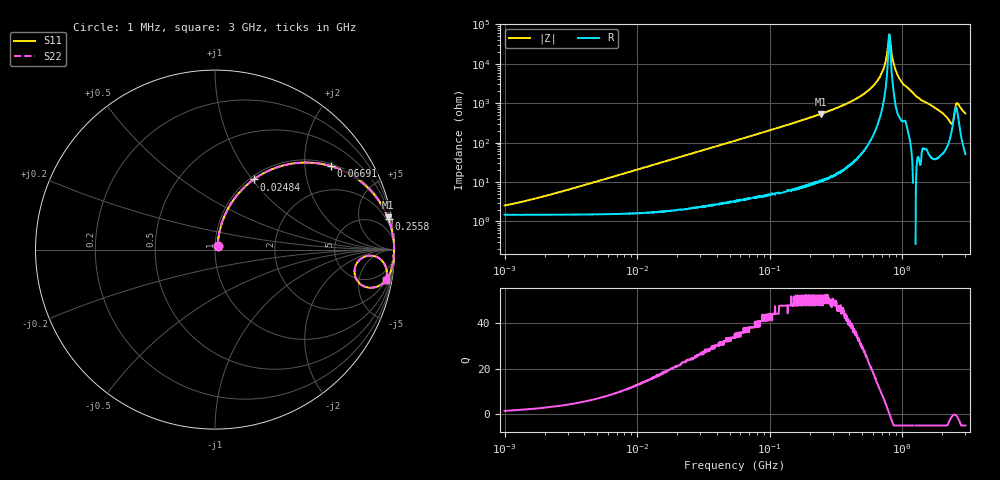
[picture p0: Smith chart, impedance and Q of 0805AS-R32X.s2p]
!s-Parameter Generated by FASTRON Sdn. Bhd.
!FASTRON P/N : 0805AS-R32X
!Keysight Technologies: E4991B_MY54100416_A.01.15
!Date: Mon Jun 15 12:54:03 2026
!Version  :Rev01  Mon Jun 15 12:54:03 2026
!Data & Calibration Information:
!Freq  S11  S21  S12  S22
!PortZ  Port1:50+j0  Port2:50+j0
!When reading reference impedance value at option line is always used.
! Remarks : This data is being provided solely for informational purposes.
# Hz S dB R 50
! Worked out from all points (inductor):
!   1601 points, 1 MHz to 3 GHz, reference 50 ohm
!   read as one part in series: L = 328 nH near 2.161 MHz
!   highest Q = 52.1 at 243.3 MHz (marker M1), where L = 348 nH
!   self-resonance near 796.6 MHz
!   S11 on the Smith chart (normalised r, x): 1 MHz: 1.03, +0.04; 24.84 MHz: 1.04, +1.02; 66.91 MHz: 1.07, +2.73; 255.8 MHz: 1, +11; 3 GHz: 2, -11
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1000000  -32.00 53.3  -0.13 -1.2  -0.13 -1.2  -32.00 53.3
3804036  -22.10 74.8  -0.15 -4.4  -0.15 -4.4  -22.10 74.8
1.447069e7  -11.00 70.4  -0.51 -16.3  -0.51 -16.3  -11.00 70.4
2.484248e7  -7.01 61.1  -1.14 -26.5  -1.14 -26.5  -7.01 61.1
5.504702e7  -2.67 41.0  -3.66 -47.3  -3.66 -47.3  -2.67 41.0
6.690963e7  -1.98 35.7  -4.67 -52.7  -4.67 -52.7  -1.98 35.7
2.083556e8  -0.25 12.6  -13.20 -76.3  -13.20 -76.3  -0.25 12.6
2.433181e8  -0.18 10.6  -14.70 -78.3  -14.70 -78.3  -0.18 10.6
2.558035e8  -0.16 10.0  -15.20 -78.9  -15.20 -78.9  -0.16 10.0
4.369573e8  -0.05 4.6  -21.90 -83.8  -21.90 -83.8  -0.05 4.6
5.988949e8  -0.02 2.1  -28.50 -84.8  -28.50 -84.8  -0.02 2.1
7.135306e8  -0.02 0.9  -36.40 -81.9  -36.40 -81.9  -0.02 0.9
7.925923e8  -0.02 0.1  -53.10 -34.7  -53.10 -34.7  -0.02 0.1
8.167498e8  -0.02 -0.2  -49.80 55.3  -49.80 55.3  -0.02 -0.2
8.71647e8  -0.02 -0.6  -39.00 79.5  -39.00 79.5  -0.02 -0.6
9.443041e8  -0.02 -1.3  -33.00 82.7  -33.00 82.7  -0.02 -1.3
1.274982e9  -0.02 -3.8  -23.60 85.7  -23.60 85.7  -0.02 -3.8
1.990301e9  -0.25 -9.6  -15.50 75.4  -15.50 75.4  -0.25 -9.6
2.301132e9  -1.23 -13.9  -11.60 53.0  -11.60 53.0  -1.23 -13.9
2.39512e9  -2.09 -8.8  -11.90 28.3  -11.90 28.3  -2.09 -8.8
2.607784e9  -0.54 -4.3  -20.50 48.0  -20.50 48.0  -0.54 -4.3
3e9  -0.28 -10.1  -15.10 74.6  -15.10 74.6  -0.28 -10.1
